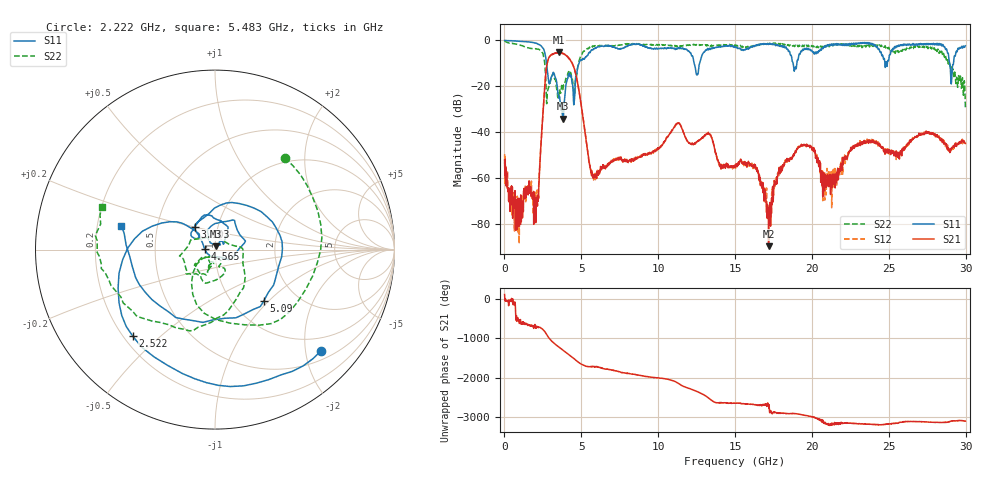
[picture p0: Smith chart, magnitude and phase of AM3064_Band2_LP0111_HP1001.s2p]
# Hz S DB R 50.0
!freq dBS11 angS11 dBS21 angS21 dBS12 angS12 dBS22 angS22
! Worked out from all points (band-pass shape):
!   1600 points, 10 MHz to 29.98 GHz, reference 50 ohm
!   highest |S21| = -5.25 dB at 3.534 GHz (marker M1); lowest = -89.6 dB at 17.18 GHz (marker M2)
!   |S21| within 3 dB of the highest: 2.849 GHz to 4.253 GHz (1.404 GHz wide, 39.5 % of centre)
!   lowest |S11| = -34.1 dB at 3.815 GHz (marker M3), VSWR 1.04, Z = 50.3 + j1.96 ohm
!   |S11| at or under -10 dB: 2.736 GHz to 4.843 GHz (2.107 GHz wide, 55.6 % of centre); 12.34 GHz to 12.69 GHz (355.9 MHz wide, 2.84 % of centre); 28.95 GHz to 29.2 GHz (255 MHz wide, 0.877 % of centre)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
!   |S22| runs from -29.2 to -0.2 dB; largest |S21 - S12| = 0.018
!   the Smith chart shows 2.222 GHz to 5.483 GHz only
!   S11 on the Smith chart (normalised r, x): 2.222 GHz: 0.69, -2.32; 2.522 GHz: 0.24, -0.41; 3.103 GHz: 0.77, +0.20; 4.565 GHz: 0.89, +0.01; 5.09 GHz: 1.37, -0.94; 5.483 GHz: 0.30, +0.11
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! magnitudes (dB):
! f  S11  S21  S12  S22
! 10 MHz  0.0  -52.2  -49.6  -0.2
! 853.5 MHz  -0.3  -78.4  -83.0  -1.8
! 2.222 GHz  -1.8  -68.8  -63.5  -3.8
! 2.522 GHz  -3.5  -29.6  -29.6  -6.2
! 3.103 GHz  -15.4  -6.0  -6.2  -15.2
! 3.534 GHz  -25.1  -5.3  -5.4  -24.4
! 3.815 GHz  -34.1  -5.7  -5.7  -20.5
! 4.565 GHz  -24.8  -12.7  -12.7  -23.5
! 5.015 GHz  -8.7  -29.2  -29.2  -6.2
! 5.09 GHz  -8.1  -32.7  -32.6  -5.3
! 5.483 GHz  -5.4  -51.7  -52.4  -3.4
! 10 GHz  -3.6  -46.8  -47.0  -2.0
! 11.31 GHz  -3.1  -36.2  -36.1  -2.6
! 15 GHz  -2.7  -54.6  -54.6  -2.1
! 16.34 GHz  -2.4  -54.9  -56.0  -2.4
! 17.18 GHz  -1.8  -89.6  -74.2  -1.6
! 18.23 GHz  -3.2  -53.4  -53.8  -1.7
! 19.99 GHz  -4.4  -46.7  -46.7  -2.2
! 20.82 GHz  -2.7  -65.4  -57.2  -2.5
! 25 GHz  -8.5  -48.5  -48.4  -3.0
! 28.31 GHz  -1.9  -42.7  -42.7  -4.6
! 29.98 GHz  -2.4  -44.9  -44.7  -29.2
